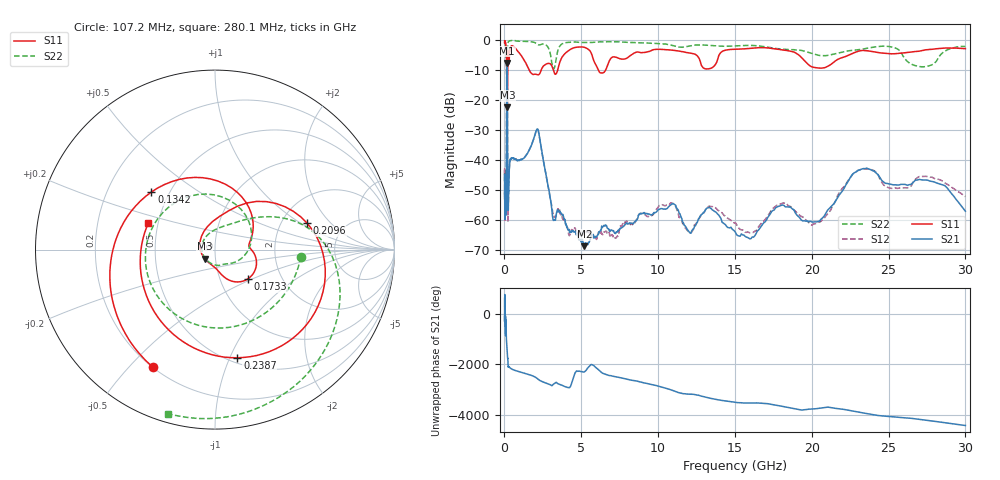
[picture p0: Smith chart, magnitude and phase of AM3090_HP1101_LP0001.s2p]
! Date/Time: Thu, Feb 28, 2019 2:07 PM
! Network Analyzer: Agilent Technologies E8364B Rev: A.07.50.67
! Sweep from 0.010 to 30.000 GHz, 1601 Points, Sweep Type: LOG
! Power Supply: 5.022 V, 0.002 A
# Hz S DB R 50
!freq MagS11 AngS11 MagS21 AngS21 MagS12 AngS12 MagS22 AngS22
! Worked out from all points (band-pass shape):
!   1601 points, 10 MHz to 30 GHz, reference 50 ohm
!   highest |S21| = -7.65 dB at 164 MHz (marker M1); lowest = -68.6 dB at 5.206 GHz (marker M2)
!   |S21| within 3 dB of the highest: 148.2 MHz to 183.8 MHz (35.6 MHz wide, 21.4 % of centre)
!   lowest |S11| = -22.3 dB at 188.7 MHz (marker M3), VSWR 1.17, Z = 44.4 - j4.52 ohm
!   |S11| at or under -10 dB: 1.609 GHz to 2.387 GHz (777.6 MHz wide, 38.9 % of centre); 3.185 GHz to 3.462 GHz (276.7 MHz wide, 8.33 % of centre); 6.109 GHz to 6.585 GHz (476.4 MHz wide, 7.51 % of centre)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
!   |S22| runs from -22.8 to -0.1 dB; largest |S21 - S12| = 0.013
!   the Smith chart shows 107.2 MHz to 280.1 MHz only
!   S11 on the Smith chart (normalised r, x): 107.2 MHz: 0.20, -0.58; 134.2 MHz: 0.40, +0.33; 173.3 MHz: 1.36, -0.47; 209.6 MHz: 2.76, +1.14; 238.7 MHz: 0.55, -1.07; 280.1 MHz: 0.44, +0.16
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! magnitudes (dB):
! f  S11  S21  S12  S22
! 10 MHz  -0.3  -46.6  -45.0  -0.5
! 38.04 MHz  -0.4  -59.2  -58.4  -1.2
! 47.89 MHz  -0.5  -48.0  -49.3  -1.3
! 107.2 MHz  -2.6  -55.7  -58.2  -6.4
! 119.1 MHz  -3.7  -52.2  -51.3  -7.2
! 134.2 MHz  -6.4  -26.7  -26.6  -9.1
! 144.7 MHz  -10.4  -13.2  -13.1  -13.5
! 164 MHz  -12.8  -7.6  -7.6  -21.1
! 173.3 MHz  -12.2  -8.2  -8.2  -22.6
! 188.7 MHz  -22.3  -13.7  -13.7  -13.0
! 209.6 MHz  -5.5  -47.8  -47.9  -2.5
! 238.7 MHz  -4.2  -56.2  -56.7  -0.8
! 280.1 MHz  -8.0  -49.0  -47.8  -0.4
! 550.5 MHz  -2.1  -39.4  -39.3  -0.2
! 2.084 GHz  -11.4  -30.0  -29.9  -1.2
! 3.204 GHz  -10.3  -60.0  -58.9  -9.6
! 5.206 GHz  -2.4  -68.6  -64.3  -0.8
! 7.926 GHz  -6.1  -61.0  -60.3  -0.8
! 15.81 GHz  -2.9  -65.7  -63.9  -1.8
! 20.41 GHz  -9.3  -60.4  -60.5  -5.0
! 23.48 GHz  -3.5  -42.8  -42.9  -2.9
! 30 GHz  -2.8  -57.0  -52.1  -2.1
